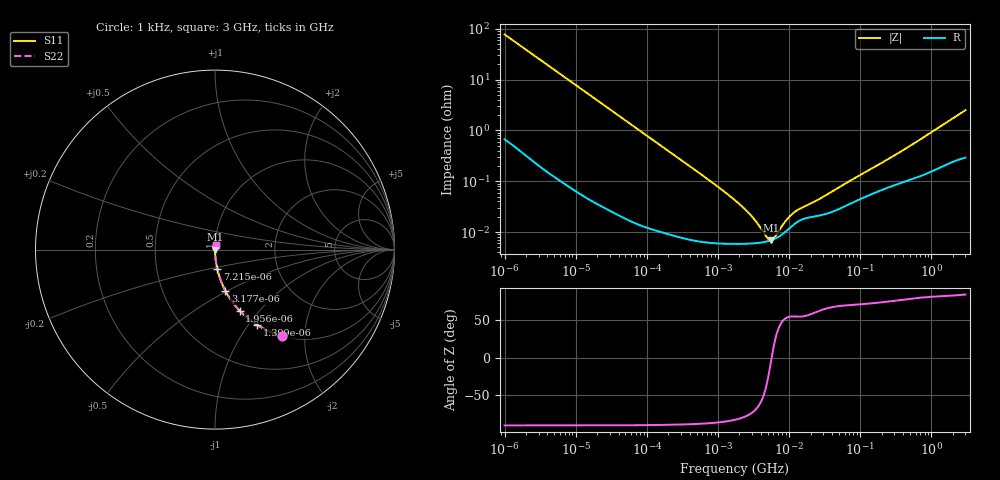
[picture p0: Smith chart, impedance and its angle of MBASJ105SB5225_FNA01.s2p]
! MBASJ105SB5225_FNA01  S-PARAMETER MODEL  ( Standard Model )
! Model Generated by TAIYO YUDEN Corporation (http://www.ty-top.com)
! Version 2.0
! TAIYO YUDEN Control No. 240725
! Copyright(c) 2013 TAIYO YUDEN CO.,LTD. All Rights Reserved.
! Product Description (link to TY-COMPAS)
! https://ds.yuden.co.jp/TYCOMPAS/or/detail?pn=MBASJ105SB5225KFNA01&u=M
! Products Name : Multilayer Ceramic Capacitors
! Characteristics :
!  Capacitance : 2.2 [uF] , Rated Voltage : 6.3 [V] , TCC : X5R
!  Case Size : 1.0 x 0.5 / 0.039 x 0.02 [mm/inch] , Thickness : 0.5 / 0.02 [mm/inch]
!  (Conditions: Temperature = 25 [degC] , DC Bias Voltage = 0 [V])
! External Node Assignments :
!  1  o---| |---o  2
! GND o---------o GND
! Frequency Range : 1kHz  -  3GHz  [ 401 STEP ]
# MHZ S RI R 50
! Freq[MHz].  S11 Real  S11 Imag  S21 Real  S21 Imag  S12 Real  S12 Imag  S22 Real  S22 Imag
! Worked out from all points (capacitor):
!   401 points, 1 kHz to 3 GHz, reference 50 ohm
!   read as one part in series: C = 2.06 uF near 1.077 kHz
!   lowest |Z| = 6.91 mohm at 5.502 MHz (marker M1)
!   series resonance near 5.673 MHz, so ESL is about 380 pH
!   S11 on the Smith chart (normalised r, x): 1 kHz: 1.01, -1.54; 1.399 kHz: 1.01, -1.10; 1.956 kHz: 1.01, -0.79; 3.177 kHz: 1.00, -0.49; 7.215 kHz: 1.00, -0.22; 3 GHz: 1.01, +0.05
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0.001  0.3733 -0.4794  0.6267 0.4794  0.6267 0.4794  0.3733 -0.4794
0.001399  0.2353 -0.4199  0.7647 0.4199  0.7647 0.4199  0.2353 -0.4199
0.001956  0.1372 -0.3399  0.8628 0.3399  0.8628 0.3399  0.1372 -0.3399
0.003177  0.0578 -0.2295  0.9422 0.2295  0.9422 0.2295  0.0578 -0.2295
0.007215  0.0123 -0.1064  0.9877 0.1064  0.9877 0.1064  0.0123 -0.1064
0.01216  0.00462 -0.0638  0.9954 0.0638  0.9954 0.0638  0.00462 -0.0638
0.033275  0.000798 -0.0235  0.9992 0.0235  0.9992 0.0235  0.000798 -0.0235
0.147855  0.000131 -0.00534  0.9999 0.00534  0.9999 0.00534  0.000131 -0.00534
0.762639  6.25e-05 -0.00103  0.9999 0.00103  0.9999 0.00103  6.25e-05 -0.00103
1.732051  5.86e-05 -0.000419  0.9999 0.000419  0.9999 0.000419  5.86e-05 -0.000419
2.812335  5.94e-05 -0.000216  0.9999 0.000216  0.9999 0.000216  5.94e-05 -0.000216
4.238263  6.28e-05 -8.44e-05  0.9999 8.44e-05  0.9999 8.44e-05  6.28e-05 -8.44e-05
4.566395  6.41e-05 -6.25e-05  0.9999 6.25e-05  0.9999 6.25e-05  6.41e-05 -6.25e-05
5.502215  6.86e-05 -8.75e-06  0.9999 8.75e-06  0.9999 8.75e-06  6.86e-05 -8.75e-06
6.881678  7.87e-05 5.56e-05  0.9999 -5.56e-05  0.9999 -5.56e-05  7.87e-05 5.56e-05
7.414467  8.38e-05 7.71e-05  0.9999 -7.71e-05  0.9999 -7.71e-05  8.38e-05 7.71e-05
9.625639  0.000112 0.000151  0.9999 -0.000151  0.9999 -0.000151  0.000112 0.000151
11.59828  0.00014 0.000196  0.9999 -0.000196  0.9999 -0.000196  0.00014 0.000196
13.97519  0.000168 0.000232  0.9998 -0.000232  0.9998 -0.000232  0.000168 0.000232
21.06097  0.000199 0.000319  0.9998 -0.000319  0.9998 -0.000319  0.000199 0.000319
256.0921  0.000772 0.0027  0.9992 -0.0027  0.9992 -0.0027  0.000772 0.0027
3000  0.00352 0.0246  0.9965 -0.0246  0.9965 -0.0246  0.00352 0.0246
